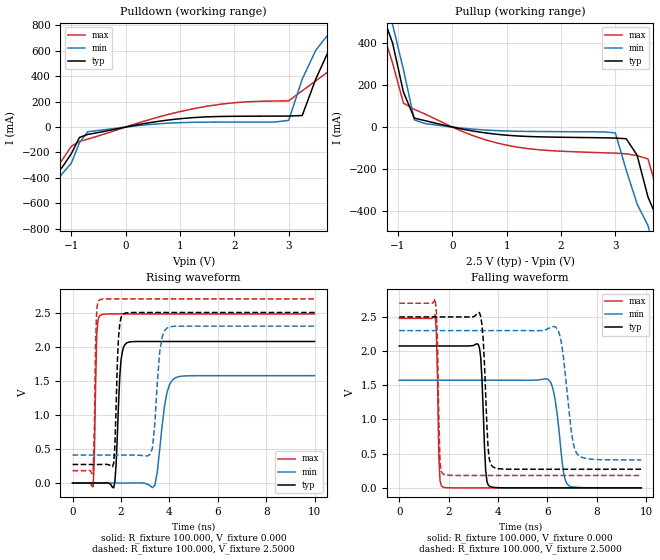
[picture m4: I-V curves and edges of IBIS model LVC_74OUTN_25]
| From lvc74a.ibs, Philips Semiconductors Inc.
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|   Model LVC_74OUTN_25
[Model]   LVC_74OUTN_25
Model_type   Output
Polarity   Non-Inverting
Vmeas =   1.25000V
Cref  =  50.0000pF
Rref  =   0.5000k
Vref  =   0.000V
C_comp   3.12pF   2.70pF   3.69pF
[Model Spec]
| Note: The input and output voltage ratings may be exceeded if the input and
|   output current ratings are observed (please refer to the data sheet)
|   Subparameter   typ   min   max
| Timing Thresholds
Vmeas   1.25   1.15   1.5
|Ambient temperature:   25.0000   85.0000   -40.0000
[Temperature Range]   35.0000   95.0000   -30.0000
[Voltage Range]   2.5000V   2.3000V   2.7000V
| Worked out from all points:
|   slope of the pulldown table from 0 to 0.375 V, typ, clamps not added: 12.6 ohm
|   slope of the pullup table from 0 to 0.375 V, typ, clamps not added: 20.2 ohm
|   rising waveform, R_fixture 100.000, V_fixture 0.000: 20-80 % time 155ps typ, 320ps min, 81.2ps max; typ from 0 V to 2.08 V
|   rising waveform, R_fixture 100.000, V_fixture 2.5000: 20-80 % time 125ps typ, 226ps min, 72.9ps max; typ from 0.272 V to 2.5 V
|   falling waveform, R_fixture 100.000, V_fixture 0.000: 20-80 % time 139ps typ, 296ps min, 76.4ps max; typ from 2.08 V to 0 V
|   falling waveform, R_fixture 100.000, V_fixture 2.5000: 20-80 % time 162ps typ, 342ps min, 86.9ps max; typ from 2.5 V to 0.272 V
|Process Range   nominal   slow   fast
[Pulldown]
| voltage   I(typ)   I(min)   I(max)
-5.5V     -4.799A    -4.734A    -4.501A
-1.75V    -814mA     -856.8mA   -764.2mA
-1.3V     -390.7mA   -435.2mA   -340.4mA
-850mV    -81.4mA    -123mA     -112.1mA
-700mV    -58.27mA   -37.32mA   -95.26mA
200mV     16.69mA    10.05mA    27.75mA
3V        86.6mA     52.68mA    206.7mA
3.25V     91mA       377.6mA    285.4mA
3.75V     613.8mA    741.2mA    442.7mA
4V        770.2mA    946.7mA    688.1mA
4.25V     1.002A     1.194A     872.6mA
11V       7.614A     7.844A     7.398A
[Pullup]
| voltage   I(typ)   I(min)   I(max)
-8.7V     7.799A     7.837A     7.764A
-1.5V     656.4mA    713.2mA    592mA
-1.3V     543.6mA    611.5mA    467mA
-1.1V     399.2mA    486.5mA    303.6mA
-900mV    166.1mA    272.9mA    113.6mA
-700mV    42.51mA    34.1mA     84.13mA
1V        -38.66mA   -18.69mA   -85.87mA
3V        -52.12mA   -27.61mA   -123.7mA
3.4V      -133.2mA   -364.8mA   -135.4mA
3.6V      -331.1mA   -467.1mA   -151.1mA
4V        -646.9mA   -851.9mA   -476.4mA
8.2V      -5.015A    -5.15A     -4.97A
[Ramp]
| variable   typ   min   max
dV/dt_r   1.245V/155.148ps   944.221mV/319.804ps   1.487V/81.173ps
dV/dt_f   1.337V/161.646ps   1.135V/342.382ps   1.511V/86.816ps
R_load = 100.000
[Rising Waveform]
R_fixture   = 100.000
V_fixture   = 0.000
V_fixture_min = 0.000
V_fixture_max = 0.000
| time   V(typ)   V(min)   V(max)
0s        41.03pV    1.687nV    3.182pV
850ps     -26.98uV   5.223uV    -55.2mV
1ns       -46.38uV   -3.16uV    2.182V
1.15ns    -124.2uV   -4.552uV   2.459V
1.75ns    22.52mV    -17.73uV   2.479V
2ns       1.794V     -42.95uV   2.479V
2.25ns    2.056V     -76.76uV   2.479V
3.4ns     2.075V     -32.37mV   2.479V
4.2ns     2.075V     1.532V     2.479V
10ns      2.075V     1.574V     2.479V
[Rising Waveform]
R_fixture   = 100.000
V_fixture   = 2.5000
V_fixture_min = 2.3000
V_fixture_max = 2.7000
| time   V(typ)   V(min)   V(max)
0s        272mV      409mV      181.2mV
850ps     271.9mV    409mV      156mV
1ns       272mV      409mV      2.553V
1.1ns     272mV      409mV      2.681V
1.7ns     289.8mV    409mV      2.7V
1.9ns     2.14V      409.1mV    2.7V
2.1ns     2.478V     409.2mV    2.7V
3.3ns     2.5V       510.4mV    2.7V
3.9ns     2.5V       2.271V     2.7V
10ns      2.5V       2.3V       2.7V
[Falling Waveform]
R_fixture   = 100.000
V_fixture   = 0.000
V_fixture_min = 0.000
V_fixture_max = 0.000
| time   V(typ)   V(min)   V(max)
0s        2.075V     1.574V     2.479V
1.45ns    2.075V     1.574V     2.53V
1.6ns     2.075V     1.574V     484.3mV
1.75ns    2.075V     1.574V     16.05mV
3.25ns    2.045V     1.574V     -5.751nV
3.5ns     252mV      1.574V     2.912nV
3.65ns    24.73mV    1.574V     3.061nV
6.1ns     11.94nV    1.56V      33.62pV
6.85ns    2.157nV    36.97mV    20.85pV
9.8ns     95.24pV    2.959uV    5.823pV
[Falling Waveform]
R_fixture   = 100.000
V_fixture   = 2.5000
V_fixture_min = 2.3000
V_fixture_max = 2.7000
| time   V(typ)   V(min)   V(max)
0s        2.5V       2.3V       2.7V
1.45ns    2.5V       2.3V       2.764V
1.65ns    2.5V       2.3V       381.2mV
1.8ns     2.5V       2.3V       196.8mV
3.25ns    2.561V     2.3V       181.2mV
3.6ns     571.8mV    2.3V       181.2mV
3.8ns     305.6mV    2.3V       181.2mV
6.35ns    272mV      2.347V     181.2mV
7.2ns     272mV      499.1mV    181.2mV
9.8ns     272mV      409mV      181.2mV
